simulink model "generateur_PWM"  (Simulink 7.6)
settings: Solver=ode15s  StartTime=0.0  StopTime=6  RelTol=1e-3
StopFcn:
  | close all, clc
  | load signal_PWM.mat
  | plot(x(1,:),x(2,:))
  | title('Signal PWM')
  | xlabel('temps')
  | grid
libraries: fl_lib x16, elec_lib x9, nesl_utility x7

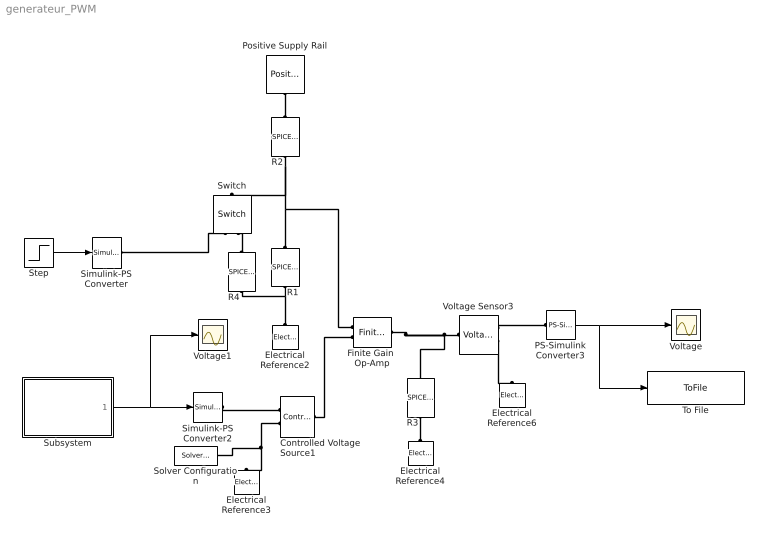
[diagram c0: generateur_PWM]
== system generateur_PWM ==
  Controlled Voltage Source1 : fl_lib/Electrical/Electrical Sources/Controlled Voltage Source  DialogController=NetworkEngine.DynNeDlgSource  SystemSampleTime=-1  i_Log=off  v_Log=off  LocalVarNames=|current|voltage|power  LocalVarDescs=|Current (A)|Voltage (V)|Power (W)  LocalVarLogging=[0 0 0]
  Electrical Reference{2..4,6} (4 alike) : fl_lib/Electrical/Electrical Elements/Electrical Reference  DialogController=NetworkEngine.DynNeDlgSource  SystemSampleTime=-1  i_Log=off  LocalVarNames=|i  LocalVarDescs=|i  LocalVarLogging=[]
  Finite Gain  Op-Amp : elec_lib/Integrated Circuits/Finite Gain Op-Amp  DialogController=NetworkEngine.DynNeDlgSource  SystemSampleTime=-1  A=1000  Rin=1e+06 Ohm  Rout=100 Ohm  Vmin=-12 V  Vmax=12 V  LocalVarNames=|power  LocalVarDescs=|Dissipated power (W)  LocalVarLogging=0
  PS-Simulink Converter3 : nesl_utility/PS-Simulink Converter  DialogController=NetworkEngine.DynNeUtilDlgSource  SystemSampleTime=-1  PhysicalDomain=network_engine_domain  LeftPortType=input  RightPortType=output  SubClassName=ps_output  Unit=1  AffineConversion=off
  Positive Supply Rail : elec_lib/Sources/Positive Supply Rail  DialogController=NetworkEngine.DynNeDlgSource  SystemSampleTime=-1  v0=15 V  current_Log=off  voltage_Log=off  power_Log=off  LocalVarNames=|current|voltage|power  LocalVarDescs=|Current (A)|Voltage (V)|Power (W)  LocalVarLogging=[0 0 0]
  R1 : elec_lib/Additional Components/SPICE-Compatible Components/Passive Devices/SPICE Resistor  DialogController=NetworkEngine.DynNeDlgSource  SystemSampleTime=-1  SCALE=1  R_param=1  R=10e3 Ohm  RSH=0 Ohm  LENGTH=1e-06 m  WIDTH=1e-06 m  NARROW=0 m  T_param=1  TC1=0 1/K  TC2=0 1/K^2  TOFFSET=0 K  TFIXED=300.15 K  TMEAS=300.15 K  LocalVarLogging=[]
  R2 : elec_lib/Additional Components/SPICE-Compatible Components/Passive Devices/SPICE Resistor  DialogController=NetworkEngine.DynNeDlgSource  SystemSampleTime=-1  SCALE=1  R_param=1  R=1e3 Ohm  RSH=0 Ohm  LENGTH=1e-06 m  WIDTH=1e-06 m  NARROW=0 m  T_param=1  TC1=0 1/K  TC2=0 1/K^2  TOFFSET=0 K  TFIXED=300.15 K  TMEAS=300.15 K  LocalVarLogging=[]
  R3 : elec_lib/Additional Components/SPICE-Compatible Components/Passive Devices/SPICE Resistor  DialogController=NetworkEngine.DynNeDlgSource  SystemSampleTime=-1  SCALE=1  R_param=1  R=10e3 Ohm  RSH=0 Ohm  LENGTH=1e-06 m  WIDTH=1e-06 m  NARROW=0 m  T_param=1  TC1=0 1/K  TC2=0 1/K^2  TOFFSET=0 K  TFIXED=300.15 K  TMEAS=300.15 K  LocalVarLogging=[]
  R4 : elec_lib/Additional Components/SPICE-Compatible Components/Passive Devices/SPICE Resistor  DialogController=NetworkEngine.DynNeDlgSource  SystemSampleTime=-1  SCALE=1  R_param=1  R=1e3 Ohm  RSH=0 Ohm  LENGTH=1e-06 m  WIDTH=1e-06 m  NARROW=0 m  T_param=1  TC1=0 1/K  TC2=0 1/K^2  TOFFSET=0 K  TFIXED=300.15 K  TMEAS=300.15 K  LocalVarLogging=[]
  Simulink-PS Converter : nesl_utility/Simulink-PS Converter  DialogController=NetworkEngine.DynNeUtilDlgSource  SystemSampleTime=-1  PhysicalDomain=network_engine_domain  LeftPortType=input  RightPortType=output  SubClassName=ps_input  Unit=1  AffineConversion=off  InputFilterTimeConstant=.001  UdotUserProvided=0
  Simulink-PS Converter2 : nesl_utility/Simulink-PS Converter  DialogController=NetworkEngine.DynNeUtilDlgSource  SystemSampleTime=-1  PhysicalDomain=network_engine_domain  LeftPortType=input  RightPortType=output  SubClassName=ps_input  Unit=1  AffineConversion=off  InputFilterTimeConstant=.001  UdotUserProvided=0
  Solver Configuration : nesl_utility/Solver Configuration  DialogController=NetworkEngine.DynNeUtilDlgSource  SystemSampleTime=-1  PhysicalDomain=network_engine_domain  LeftPortType=input  RightPortType=generic  SubClassName=solver  Accelerate=off  Profile=off  ResidualTolerance=1e-12  MaxNonlinIter=12  MaxModeIter=2  DoFixedCost=on  UseLocalSampling=off  DoDC=off  LinearAlgebra=Sparse  LocalSolverSampleTime=.001  LocalSolverChoice=NE_BACKWARD_EULER_ADVANCER  UseLocalSolver=off
  Step : Step  Time=3  Before=1  After=0  SampleTime=0
  Subsystem : Subsystem
  Switch : fl_lib/Electrical/Electrical Elements/Switch  DialogController=NetworkEngine.DynNeDlgSource  SystemSampleTime=-1  R_closed=0.01 Ohm  G_open=1e-08 1/Ohm  Threshold=0  i_Log=off  v_Log=off  LocalVarNames=|i|v  LocalVarDescs=|i|v  LocalVarLogging=[0 0]
  To File : ToFile  Filename=signal_PWM  MatrixName=x
  Voltage : Scope
  Voltage Sensor3 : fl_lib/Electrical/Electrical Sensors/Voltage Sensor  DialogController=NetworkEngine.DynNeDlgSource  SystemSampleTime=-1  i1_Log=off  v1_Log=off  LocalVarNames=|i1|v1  LocalVarDescs=|i1|v1  LocalVarLogging=[]
  Voltage1 : Scope
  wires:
  PS-Simulink Converter3/1 -> Voltage/1, To File/1
  Subsystem/1(Out1) -> Simulink-PS Converter2/1, Voltage1/1
  Step/1 -> Simulink-PS Converter/1
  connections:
  R2/LConn1 -- R1/RConn1 -- Finite Gain  Op-Amp/LConn1 -- Switch/LConn1
  Simulink-PS Converter2/RConn1 -- Controlled Voltage Source1/RConn1
  Controlled Voltage Source1/LConn1 -- Finite Gain  Op-Amp/LConn2
  Electrical Reference4/LConn1 -- R3/LConn1
  Voltage Sensor3/RConn1 -- PS-Simulink Converter3/LConn1
  Finite Gain  Op-Amp/RConn1 -- R3/RConn1 -- Voltage Sensor3/LConn1
  Voltage Sensor3/RConn2 -- Electrical Reference6/LConn1
  Controlled Voltage Source1/RConn2 -- Electrical Reference3/LConn1 -- Solver Configuration/RConn1
  Positive Supply Rail/RConn1 -- R2/RConn1
  Simulink-PS Converter/RConn1 -- Switch/RConn1
  R4/LConn1 -- R1/LConn1 -- Electrical Reference2/LConn1
  R4/RConn1 -- Switch/RConn2

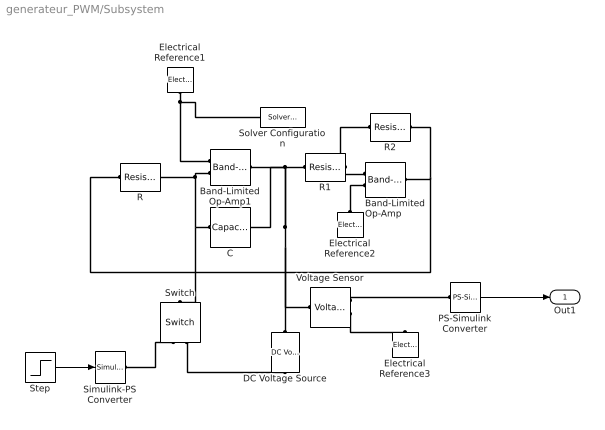
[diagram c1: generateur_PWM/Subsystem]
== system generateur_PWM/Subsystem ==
  Band-Limited Op-Amp : elec_lib/Integrated Circuits/Band-Limited Op-Amp  DialogController=NetworkEngine.DynNeDlgSource  SystemSampleTime=-1  A=1000  Rin=1e+06 Ohm  Rout=100 Ohm  Vmin=-15 V  Vmax=15 V  Vdotmax=1000 V/s  f=1e+05 Hz  V0=0 V  LocalVarNames=|power  LocalVarDescs=|Dissipated power (W)  LocalVarLogging=0
  Band-Limited Op-Amp1 : elec_lib/Integrated Circuits/Band-Limited Op-Amp  DialogController=NetworkEngine.DynNeDlgSource  SystemSampleTime=-1  A=1000  Rin=1e+06 Ohm  Rout=100 Ohm  Vmin=-15 V  Vmax=15 V  Vdotmax=1000 V/s  f=1e+05 Hz  V0=0 V  LocalVarNames=|power  LocalVarDescs=|Dissipated power (W)  LocalVarLogging=0
  C : fl_lib/Electrical/Electrical Elements/Capacitor  DialogController=NetworkEngine.DynNeDlgSource  SystemSampleTime=-1  c=1e-6 F  v0=0 V  r=1e-6 Ohm  g=0 1/Ohm  i_Log=off  v_Log=off  vc_Log=off  LocalVarNames=|current|voltage|power  LocalVarDescs=|Capacitor current (A)|Voltage across capacitor (V)|Power (W)  LocalVarLogging=[0 0 0]
  DC Voltage Source : elec_lib/Additional Components/SPICE-Compatible Components/Sources/DC Voltage Source  DialogController=NetworkEngine.DynNeDlgSource  SystemSampleTime=-1  DC=1 V  current_Log=off  voltage_Log=off  power_Log=off  LocalVarNames=|current|voltage|power  LocalVarDescs=|Current (A)|Voltage (V)|Power (W)  LocalVarLogging=[0 0 0]
  Electrical Reference1 : fl_lib/Electrical/Electrical Elements/Electrical Reference  DialogController=NetworkEngine.DynNeDlgSource  SystemSampleTime=-1  i_Log=off  LocalVarNames=|i  LocalVarDescs=|i  LocalVarLogging=[]
  Electrical Reference2 : fl_lib/Electrical/Electrical Elements/Electrical Reference  DialogController=NetworkEngine.DynNeDlgSource  SystemSampleTime=-1  i_Log=off  LocalVarNames=|i  LocalVarDescs=|i  LocalVarLogging=[]
  Electrical Reference3 : fl_lib/Electrical/Electrical Elements/Electrical Reference  DialogController=NetworkEngine.DynNeDlgSource  SystemSampleTime=-1  i_Log=off  LocalVarNames=|i  LocalVarDescs=|i  LocalVarLogging=[]
  PS-Simulink Converter : nesl_utility/PS-Simulink Converter  DialogController=NetworkEngine.DynNeUtilDlgSource  SystemSampleTime=-1  PhysicalDomain=network_engine_domain  LeftPortType=input  RightPortType=output  SubClassName=ps_output  Unit=1  AffineConversion=off
  R : fl_lib/Electrical/Electrical Elements/Resistor  DialogController=NetworkEngine.DynNeDlgSource  SystemSampleTime=-1  R=100e3 Ohm  i_Log=off  v_Log=off  LocalVarNames=|current|voltage|power  LocalVarDescs=|Resistor current (A)|Voltage across resistor (V)|Power (W)  LocalVarLogging=[0 0 0]
  R1 : fl_lib/Electrical/Electrical Elements/Resistor  DialogController=NetworkEngine.DynNeDlgSource  SystemSampleTime=-1  R=10e3 Ohm  i_Log=off  v_Log=off  LocalVarNames=|current|voltage|power  LocalVarDescs=|Resistor current (A)|Voltage across resistor (V)|Power (W)  LocalVarLogging=[0 0 0]
  R2 : fl_lib/Electrical/Electrical Elements/Resistor  DialogController=NetworkEngine.DynNeDlgSource  SystemSampleTime=-1  R=10e3 Ohm  i_Log=off  v_Log=off  LocalVarNames=|current|voltage|power  LocalVarDescs=|Resistor current (A)|Voltage across resistor (V)|Power (W)  LocalVarLogging=[0 0 0]
  Simulink-PS Converter : nesl_utility/Simulink-PS Converter  DialogController=NetworkEngine.DynNeUtilDlgSource  SystemSampleTime=-1  PhysicalDomain=network_engine_domain  LeftPortType=input  RightPortType=output  SubClassName=ps_input  Unit=1  AffineConversion=off  InputFilterTimeConstant=.001  UdotUserProvided=0
  Solver Configuration : nesl_utility/Solver Configuration  DialogController=NetworkEngine.DynNeUtilDlgSource  SystemSampleTime=-1  PhysicalDomain=network_engine_domain  LeftPortType=input  RightPortType=generic  SubClassName=solver  Accelerate=off  Profile=off  ResidualTolerance=1e-9  MaxNonlinIter=12  MaxModeIter=2  DoFixedCost=off  UseLocalSampling=off  DoDC=off  LinearAlgebra=Sparse  LocalSolverSampleTime=.001  LocalSolverChoice=NE_BACKWARD_EULER_ADVANCER  UseLocalSolver=off
  Step : Step  Time=0  Before=0.1  After=0  SampleTime=0
  Switch : fl_lib/Electrical/Electrical Elements/Switch  DialogController=NetworkEngine.DynNeDlgSource  SystemSampleTime=-1  R_closed=0.01 Ohm  G_open=1e-08 1/Ohm  Threshold=0  i_Log=off  v_Log=off  LocalVarNames=|i|v  LocalVarDescs=|i|v  LocalVarLogging=[0 0]
  Voltage Sensor : fl_lib/Electrical/Electrical Sensors/Voltage Sensor  DialogController=NetworkEngine.DynNeDlgSource  SystemSampleTime=-1  i1_Log=off  v1_Log=off  LocalVarNames=|i1|v1  LocalVarDescs=|i1|v1  LocalVarLogging=[]
  Out1 : Outport
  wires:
  Step/1 -> Simulink-PS Converter/1
  PS-Simulink Converter/1 -> Out1/1
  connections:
  R1/RConn1 -- Band-Limited Op-Amp/LConn1 -- R2/LConn1
  Electrical Reference2/LConn1 -- Band-Limited Op-Amp/LConn2
  R2/RConn1 -- Band-Limited Op-Amp/RConn1 -- R/LConn1
  Electrical Reference1/LConn1 -- Band-Limited Op-Amp1/LConn1 -- Solver Configuration/RConn1
  C/LConn1 -- R/RConn1 -- Band-Limited Op-Amp1/LConn2 -- Switch/LConn1
  C/RConn1 -- Voltage Sensor/LConn1 -- DC Voltage Source/LConn1 -- Band-Limited Op-Amp1/RConn1 -- R1/LConn1
  Switch/RConn2 -- DC Voltage Source/RConn1
  Voltage Sensor/RConn2 -- Electrical Reference3/LConn1
  Voltage Sensor/RConn1 -- PS-Simulink Converter/LConn1
  Simulink-PS Converter/RConn1 -- Switch/RConn1
